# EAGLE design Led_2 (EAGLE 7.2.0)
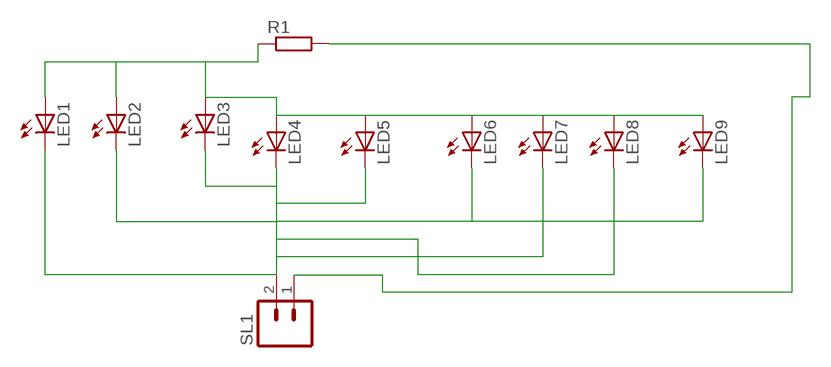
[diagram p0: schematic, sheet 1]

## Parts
LED1  LED10MM  [LED10MM]
LED2  LED10MM  [LED10MM]
LED3  LED10MM  [LED10MM]
LED4  LED10MM  [LED10MM]
LED5  LED10MM  [LED10MM]
LED6  LED10MM  [LED10MM]
LED7  LED10MM  [LED10MM]
LED8  LED10MM  [LED10MM]
LED9  LED10MM  [LED10MM]
R1  R-EU_0207/12  [0207/12]
SL1  M02  [02P]

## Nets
N$1: LED1.K(C) LED2.K(C) LED3.K(C) LED4.K(C) LED5.K(C) LED6.K(C) LED7.K(C) LED8.K(C) LED9.K(C) SL1.2
N$3: R1.2 SL1.1
N$4: LED1.A LED2.A LED3.A LED4.A LED5.A LED6.A LED7.A LED8.A LED9.A R1.1

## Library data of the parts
LED1-LED9 = led:LED: LED
R1 = rcl:R-EU_: RESISTOR, European symbol
SL1 = con-amp-quick:M02: AMP QUICK CONNECTOR; OC_FARNELL: unknown; OC_NEWARK: unknown

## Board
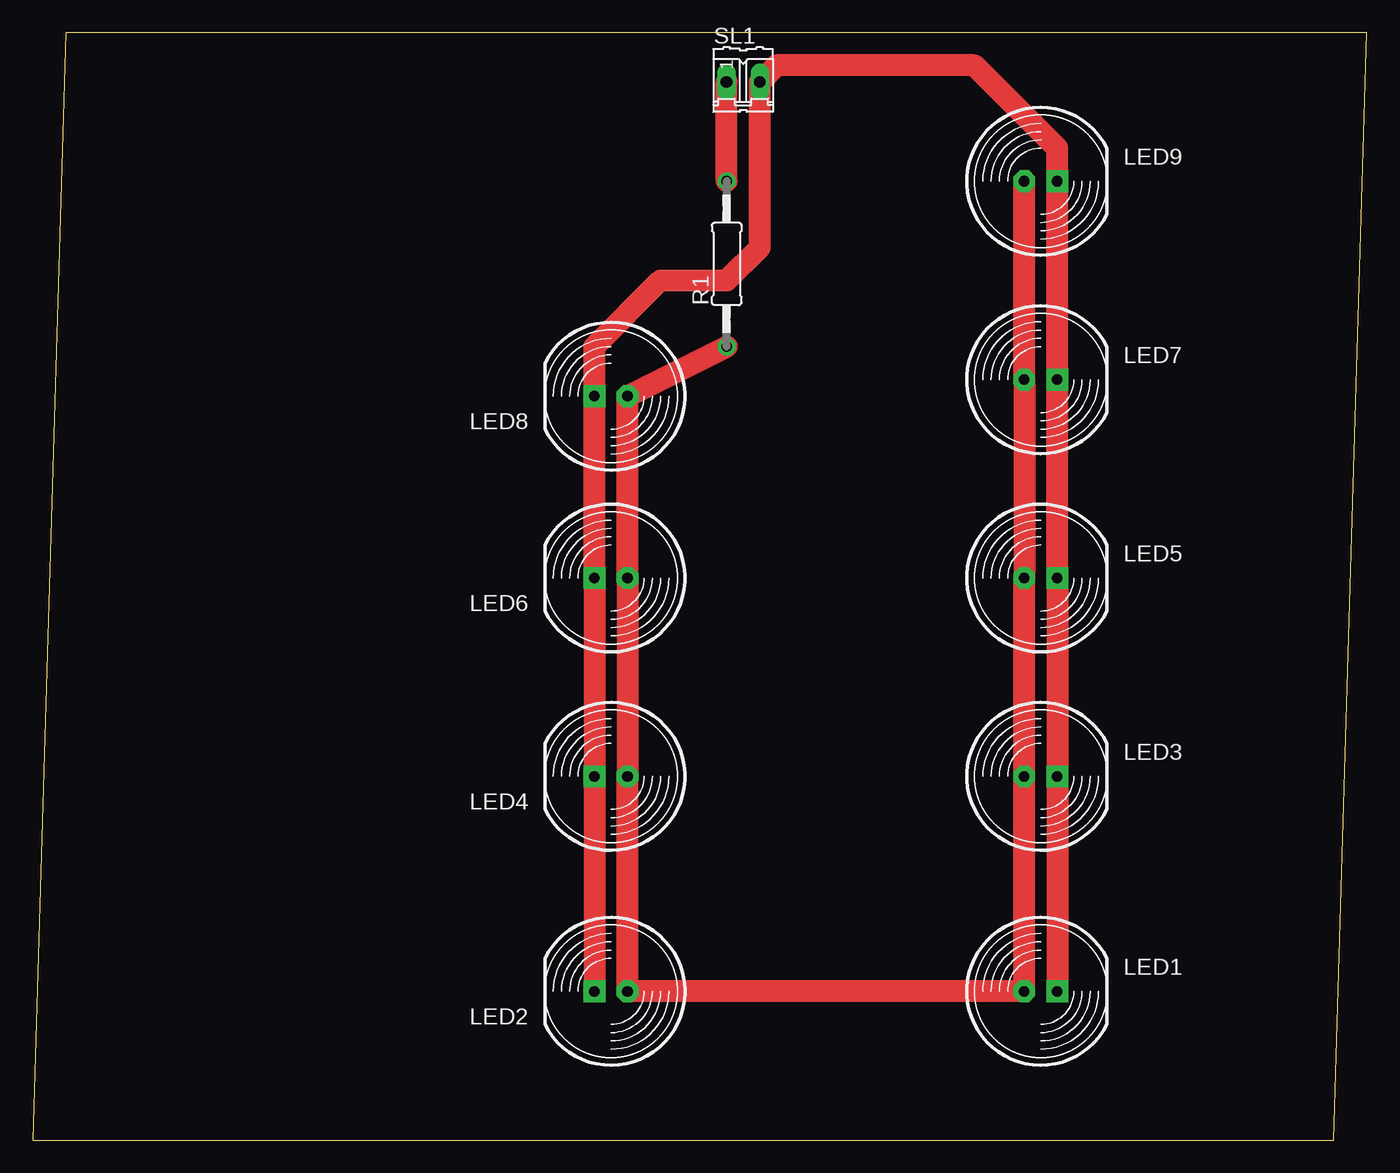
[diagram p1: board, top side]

Size 102.54 x 85.08 mm. Coordinates in mm from the lower left corner, seen from the top.
Outline: 0,0 100,0 102.54,85.08 2.54,85.08 0,0
Copper layers (1*16): Top 0.035mm / dielectric 1.5mm / Bottom 0.035mm
Design rules "default": minimum track width 10mil, minimum drill 24mil, track to track 8mil, track to pad 8mil, pad to pad 8mil, via to via 8mil, smd to smd 8mil, copper to edge 40mil, drill to drill 8mil, minimum pad ring 10mil, minimum via ring 8mil, stop-mask expansion 4mil, vias tented up to drill 0mil, thermal gap 10mil

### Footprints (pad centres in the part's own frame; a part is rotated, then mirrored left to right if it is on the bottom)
LED10MM = drill 0.813 pad 1.676 octagon: A -1.27,0 | drill 0.813 pad 1.676 square: K 1.27,0
0207/12 = drill 0.813 octagon: 1 -6.35,0; 2 6.35,0
02P = drill 0.914 long: 1 -1.27,0; 2 1.27,0

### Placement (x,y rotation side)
LED1  77.47,11.43 0 top
LED2  44.45,11.43 180 top
LED3  77.47,27.94 0 top
LED4  44.45,27.94 180 top
LED5  77.47,43.18 0 top
LED6  44.45,43.18 180 top
LED7  77.47,58.42 0 top
LED8  44.45,57.15 180 top
LED9  77.47,73.66 0 top
R1  53.34,67.31 90 top
SL1  54.61,81.28 0 top

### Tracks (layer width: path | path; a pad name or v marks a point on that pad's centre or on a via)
N$1
  Top 1.676: LED1.K LED3.K LED5.K LED7.K LED9.K 78.74,76.2 72.39,82.55 57.15,82.55 SL1.2 55.88,68.58 53.34,66.04 48.26,66.04 43.18,60.96 LED8.K LED6.K LED4.K LED2.K
N$3
  Top 1.676: R1.2 SL1.1
N$4
  Top 1.676: R1.1 LED8.A LED6.A LED4.A LED2.A LED1.A LED3.A LED5.A LED7.A LED9.A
